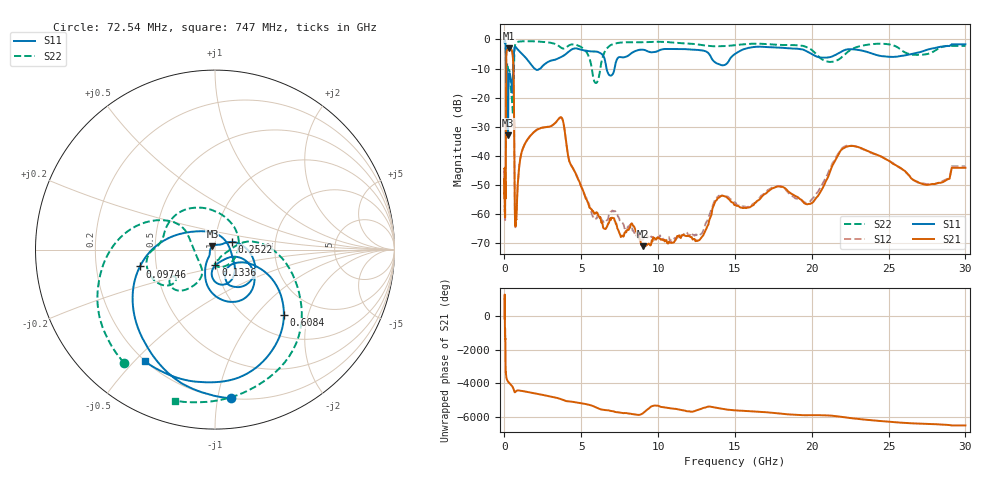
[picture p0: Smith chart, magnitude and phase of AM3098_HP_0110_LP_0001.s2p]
! Date/Time: Thu, Feb 28, 2019 8:37 AM
! Network Analyzer: Agilent Technologies E8364B Rev: A.07.50.67
! Sweep from 0.010 to 30.000 GHz, 1601 Points, Sweep Type: LOG
! Power Supply: 5.023 V, 0.002 A
# Hz S DB R 50
!freq MagS11 AngS11 MagS21 AngS21 MagS12 AngS12 MagS22 AngS22
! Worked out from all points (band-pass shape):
!   1601 points, 10 MHz to 30 GHz, reference 50 ohm
!   highest |S21| = -3.02 dB at 267.8 MHz (marker M1); lowest = -71.0 dB at 9.027 GHz (marker M2)
!   |S21| within 3 dB of the highest: 117.2 MHz to 546.3 MHz (429.1 MHz wide, 129 % of centre)
!   lowest |S11| = -32.9 dB at 231.6 MHz (marker M3), VSWR 1.05, Z = 48.6 + j1.71 ohm
!   |S11| at or under -10 dB: 175.2 MHz to 571.4 MHz (396.2 MHz wide, 106 % of centre); 1.966 GHz to 2.328 GHz (361.9 MHz wide, 16.9 % of centre); 6.643 GHz to 7.165 GHz (521.6 MHz wide, 7.55 % of centre)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
!   |S22| runs from -25.9 to -0.5 dB; largest |S21 - S12| = 0.009
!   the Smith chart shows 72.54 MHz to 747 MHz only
!   S11 on the Smith chart (normalised r, x): 72.54 MHz: 0.20, -1.09; 97.46 MHz: 0.40, -0.09; 133.6 MHz: 0.99, -0.17; 252.2 MHz: 1.21, +0.10; 608.4 MHz: 1.40, -1.42; 747 MHz: 0.20, -0.53
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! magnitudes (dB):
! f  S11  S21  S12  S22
! 10 MHz  -0.3  -44.5  -45.1  -0.5
! 38.04 MHz  -0.5  -58.4  -58.1  -0.8
! 72.54 MHz  -1.6  -52.8  -52.1  -1.8
! 84.29 MHz  -2.7  -50.9  -51.1  -2.9
! 97.46 MHz  -7.4  -23.5  -23.4  -8.7
! 133.6 MHz  -21.1  -4.4  -4.4  -11.0
! 144.7 MHz  -18.6  -3.9  -3.9  -11.2
! 186.8 MHz  -11.1  -3.6  -3.5  -8.2
! 231.6 MHz  -32.9  -3.1  -3.1  -10.0
! 252.2 MHz  -19.6  -3.1  -3.0  -10.4
! 267.8 MHz  -15.6  -3.0  -3.0  -10.6
! 550.5 MHz  -13.5  -6.3  -6.2  -25.9
! 608.4 MHz  -5.5  -16.7  -16.6  -10.5
! 682.6 MHz  -2.6  -61.5  -60.7  -2.1
! 747 MHz  -2.7  -61.9  -61.4  -1.2
! 2.084 GHz  -10.5  -31.1  -31.1  -0.7
! 3.704 GHz  -6.0  -26.8  -26.8  -2.9
! 7.926 GHz  -5.9  -66.2  -64.7  -1.0
! 9.027 GHz  -3.5  -71.0  -68.7  -0.9
! 19.8 GHz  -4.4  -56.5  -55.9  -3.0
! 22.67 GHz  -3.4  -36.6  -36.5  -3.2
! 30 GHz  -1.7  -44.1  -43.5  -2.2
